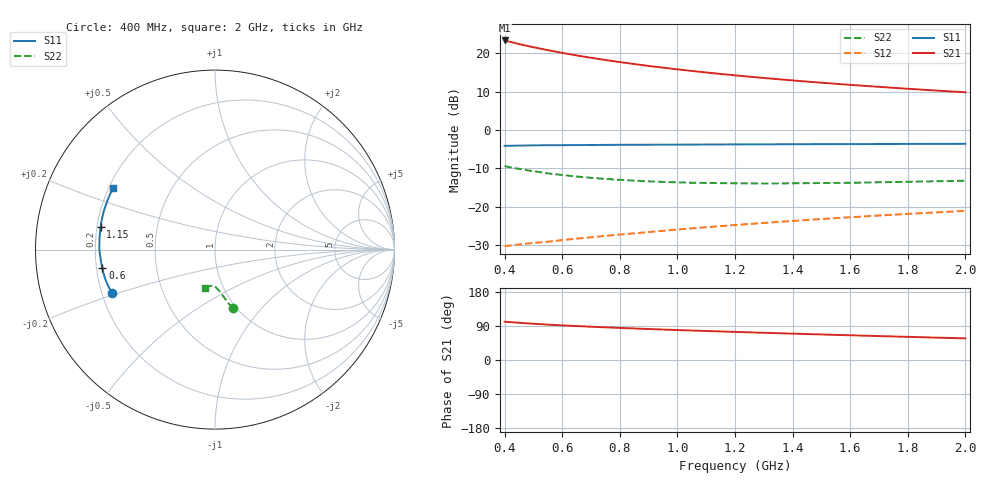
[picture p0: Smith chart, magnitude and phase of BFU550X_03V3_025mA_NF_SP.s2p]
! Filename:  P:\Prog\Test\Noise\ATS_data\Testdata_Net\bfu550X de embed 3currents\BFU550X_APG2013_44_C05_03p3V_025mA_NF_CM01_D.sf
! Date/Time: Mon 29/Jul/2013 14:56:12
! BFU550X_APG2013_44_C05_03p3V_1to35mA_NF_CM01_Bias7_R.sf
! Noise Parameter Data File
! BFU550X_APG2013_44_C05_03p3V_1to35mA_NF_CM01
! Date/time: Fri Jul 19 17:23:25 2013
! VAR V_out= 3.300000
! VAR I_out= 24.995000
! VAR V_in= 0.842000
! VAR I_in= 0.289600
! Device data file deembeded for feedlines and parallel
! Original file: \bfu550X de embed 3currents\BFU550X_APG2013_44_C05_03p3V_025mA_NF_CM01_R.sf
! Feed-files: PR005V01_100713_Feed1.s2p, PR005V01_100713_Feed2.s2p
! Parallel-file: PR005V01_100713_Par.s2p
# MHz S MA R 50
!  Freq-MHz  S11-mag  S11-arg  S21-mag  S21-arg  S12-mag  S12-arg  S22-mag  S22-arg
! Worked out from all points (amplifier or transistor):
!   37 points, 400 MHz to 2 GHz, reference 50 ohm
!   highest |S21| = 23.3 dB at 400 MHz (marker M1)
!   |S21| within 3 dB of that: start of sweep to 583.6 MHz
!   unconditionally stable (mu >= 1): 1.206 GHz to end of sweep
!   at 500 MHz: K = 0.71, MSG = 25.5 dB, |S12| = -29.4 dB
!   at 1.1 GHz: K = 0.98, MSG = 20.1 dB, |S12| = -25.3 dB
!   at 2 GHz: K = 1.06, MAG = 13.9 dB, |S12| = -21.0 dB
!   lowest NFmin = 1.09 dB at 480 MHz
!   S11 on the Smith chart (normalised r, x): 400 MHz: 0.24, -0.19; 600 MHz: 0.22, -0.08; 1.15 GHz: 0.21, +0.09; 2 GHz: 0.22, +0.27
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400  0.6246 -157.3  14.69 101.0  0.03082 47.3  0.3401 -73.1
420  0.6247 -158.9  14.05 99.9  0.03144 47.6  0.3279 -74.2
440  0.6278 -160.6  13.48 98.8  0.03212 47.9  0.317 -74.8
480  0.6308 -163.5  12.45 96.7  0.03336 48.5  0.299 -76.7
500  0.6327 -164.9  11.99 95.7  0.03393 48.7  0.2921 -77.3
550  0.6356 -168.2  10.99 93.4  0.03523 49.7  0.2731 -79.0
600  0.6359 -170.8  10.12 91.4  0.03697 50.7  0.2603 -80.4
650  0.6384 -173.3  9.376 89.6  0.03859 51.5  0.2486 -81.7
700  0.6393 -175.6  8.736 87.8  0.04025 52.3  0.2392 -83.0
750  0.6418 -177.7  8.173 86.2  0.04196 53.0  0.2315 -84.1
800  0.6438 -179.7  7.682 84.7  0.0436 53.7  0.225 -85.4
850  0.6448 178.4  7.243 83.2  0.04525 54.5  0.2196 -86.4
900  0.6449 176.6  6.849 81.8  0.04706 55.2  0.2152 -87.3
950  0.6462 175.0  6.499 80.4  0.04883 55.7  0.2115 -88.3
1050  0.6476 171.9  5.89 77.8  0.05253 56.7  0.2064 -90.2
1150  0.6498 169.0  5.386 75.3  0.05621 57.4  0.2041 -91.8
1200  0.6508 167.5  5.165 74.1  0.05808 57.7  0.203 -92.7
1350  0.6537 163.5  4.596 70.7  0.06375 58.5  0.2021 -95.2
1500  0.656 159.8  4.141 67.4  0.06948 58.8  0.2044 -97.5
1600  0.6572 157.4  3.883 65.2  0.0733 59.0  0.206 -99.0
1750  0.6593 154.0  3.551 62.1  0.07919 59.0  0.2107 -101.4
2000  0.6631 148.6  3.106 57.1  0.08882 58.8  0.2194 -105.0
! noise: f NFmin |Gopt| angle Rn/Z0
400  1.171  0.3339  -176.4  0.0735
460  1.109  0.3968  -171.3  0.0562
600  1.138  0.3636  -170.6  0.0678
800  1.139  0.412  -167.7  0.0574
1000  1.168  0.4366  -164.9  0.0549
1200  1.188  0.4432  -162.7  0.0582
1400  1.204  0.468  -158  0.0612
1600  1.244  0.4809  -153.4  0.0679
1800  1.229  0.5044  -151.4  0.0659
2000  1.271  0.541  -148.7  0.0687
